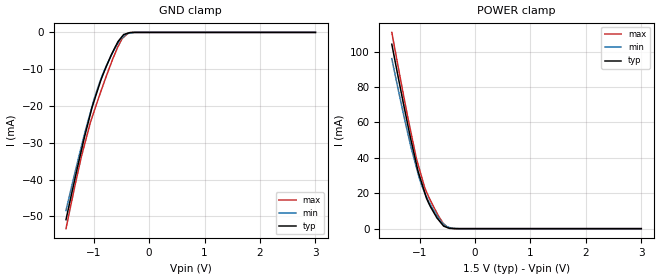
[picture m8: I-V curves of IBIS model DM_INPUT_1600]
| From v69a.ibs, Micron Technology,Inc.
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| MODEL DM_INPUT_1600 (DM Input Model with no ODT, 1600Mbps)
[Model]   DM_INPUT_1600
Model_type   Input
Vinl = 600.000mV
Vinh = 900.000mV
|   typ   min   max
C_comp   1.24pF   1.09pF   1.39pF
[Model Spec]
| Input threshold voltage corners
Vinl   0.6000V   0.5625V   0.6375V
Vinh   0.9000V   0.8625V   0.9375V
[Receiver Thresholds]
Vth   =  0.750V
Vth_min  =  0.735V
Vth_max  =  0.765V
Vinh_ac  =  0.150V
Vinh_dc  =  0.100V
Vinl_ac  = -0.150V
Vinl_dc  = -0.100V
Tslew_ac =  5.000ns |Not specified, so set to high value
[Voltage Range]   1.5000V   1.4250V   1.5750V
| Junction Temperature (Ambient temp is 35C typ, 95C min, 0C max)
[Temperature Range]   50.0   110.0   0.0
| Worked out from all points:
|   GND clamp passes 1 mA (typ) near -0.48 V on its own axis
|   POWER clamp passes 1 mA (typ) near -0.53 V on its own axis
[GND Clamp]
|   Voltage   I(typ)   I(min)   I(max)
-1.5V     -50.86mA   -48.39mA   -53.31mA
-1.335V   -39.51mA   -37.89mA   -41.36mA
-1.22V    -31.91mA   -30.85mA   -33.59mA
-1.06V    -22.14mA   -21.75mA   -24.46mA
-1.03V    -20.37mA   -20.11mA   -23.1mA
-875mV    -13.13mA   -12.88mA   -16.2mA
-765mV    -8.986mA   -8.82mA    -11.56mA
-635mV    -4.662mA   -4.732mA   -6.435mA
-565mV    -2.562mA   -2.983mA   -3.942mA
-485mV    -1.053mA   -1.384mA   -1.64mA
-380mV    -208.9uA   -292.7uA   -211uA
3V        0A         0A         0A
[POWER Clamp]
|   Voltage   I(typ)   I(min)   I(max)
-1.5V     104.2mA    96.04mA    110.8mA
-1.22V    59.88mA    55.04mA    64.17mA
-1.155V   50.11mA    46.13mA    54.38mA
-1.06V    36.99mA    35.03mA    40.06mA
-1.025V   32.28mA    30.95mA    36.2mA
-905mV    20.23mA    20.1mA     23.06mA
-800mV    12.24mA    13.34mA    15.7mA
-635mV    4.119mA    4.874mA    6.02mA
-565mV    1.438mA    2.643mA    2.719mA
-490mV    520.5uA    937.2uA    712uA
-285mV    1.423uA    9.711uA    221nA
3V        0A         0A         0A
